PROGRAM MAIN
VAR_INPUT
   // Use an external Switch to start justify Offset/Gain
   bEnable AT%I*         :BOOL;
   PAI_Sample AT%I*      :DINT; // The linked Variable to the EL3751 Result
END_VAR
VAR
   // "Main" State controlling Offset/Gain adjusting:
   nMainCal_State        :BYTE:=0;
   // ===============================================
   // For CoE Object 0x8005 access:
   fb_coe_write          :FB_EcCoESdoWrite;
   
   // Enter your Net-Id here:
   userNetId             :T_AmsNetId := 'xxx.xx.1.1.2.1';
   // Enter your EL3751 adress here:
   userSlaveAddr         :UINT := 1001;
   
   wCoEIndexScaler       :WORD := 16#8005;
   bySubIndScalGain      :BYTE := 16#02;
   bySubIndScalOffs      :BYTE := 16#01;
   nADSErrId             :UDINT; // Copy of ADS-Error ID
   // ===============================================
   // Variables for calculation
   fb_get_min_max        :FB_GET_MIN_MAX;
   // Variables used for offset scaling:
   nSTATE_SCALE_OFFSET   :INT := 0;
   bStartScaleOffset     :BOOL := FALSE;
   bScaleOffsetDone      :BOOL := FALSE;
   fOffsetDeviationVal   :REAL;
   fScalerOffset_COE     :LREAL := 0;
   wOFFSET_MIN_VAL_REF   :WORD;
   // Variables used for gain scaling:
   nSTATE_SCALE_GAIN     :INT := 0;
   bStartScaleGain       :BOOL := FALSE;
   bScaleGainDone        :BOOL := FALSE;
   fScalerGain_COE       :REAL := 1;
   nPRESET_MAX_VAL       :DINT := 3000000; // Target amplitude value
   nMaxAmplVal           :DINT;
   // ===============================================
   // Variables for intermediate results
   nValue                :DINT; // Used for Offset (adding)
   fValue                :REAL; // Used for Gain (multiply)
END_VAR

// Example program 1 and 2 program code:
// =====================================
IF bEnable AND (nMainCal_State = 0) THEN // Poll Switch
   nMainCal_State := 10; // Start
END_IF
CASE nMainCal_State OF // Main-State Procedure
   10:
      bStartScaleOffset:=TRUE; // Start with Offset scaling
      wOFFSET_MIN_VAL_REF := 2000; // Prepare deviation tolerance value scope
      nMainCal_State := nMainCal_State + 1; // next state
   11:
      IF bScaleOffsetDone THEN
         bStartScaleGain := TRUE; // Continue with gain scaling
         nMainCal_State := nMainCal_State + 1;
      END_IF
   12:
      IF bScaleGainDone THEN
         nMainCal_State := nMainCal_State + 1; // all done
      END_IF
   13:
      IF NOT bEnable THEN
         nMainCal_State :=0; // Initalization for next start by user
      END_IF
END_CASE
// ----- Offset scaling -----
IF bStartScaleOffset THEN
   CASE nSTATE_SCALE_OFFSET OF
   0:
      bScaleOffsetDone := FALSE; // Initialization of confirmation flag
      nSTATE_SCALE_OFFSET := nSTATE_SCALE_OFFSET + 1;
   1:
      fb_get_min_max(nInputValue:=PAI_Sample); // Get min/max Values by current Sample value
      IF fb_get_min_max.bRESULT THEN // Wait if Limit-Values are valid
         fb_coe_write(bExecute := FALSE); // Prepare CoE access
         nSTATE_SCALE_OFFSET := nSTATE_SCALE_OFFSET + 1; // Min/Max Values valid - go to next state
      END_IF
   2:
      // Calculate current offset deviation
      fOffsetDeviationVal :=
      LREAL_TO_REAL(ABS(fb_get_min_max.nMinVal) - ((ABS(fb_get_min_max.nMaxVal) + ABS(fb_get_min_max.nMinVal))/2));
      // Offset deviation check:
      IF ABS(fOffsetDeviationVal) < wOFFSET_MIN_VAL_REF THEN
         // Deviation in acceptable range - offset scaling done
         bScaleOffsetDone := TRUE;
         bStartScaleOffset := FALSE;
         nSTATE_SCALE_OFFSET := 0;
      ELSE
         // Calculate new offset value (consider pre-assigned value)
         nValue := LREAL_TO_DINT(fScalerOffset_COE + fOffsetDeviationVal);
         // ..proceed zero-point shift: write value into CoE Object
         fb_coe_write(
            sNetId:= userNetId,
            nSlaveAddr:= userSlaveAddr,
            nSubIndex:= bySubIndScalOffs,
            nIndex:= wCoEIndexScaler,
            pSrcBuf:= ADR(nValue), // Offset-Value (CoE 0x8005:01)
            cbBufLen:= SIZEOF(nValue),
            bExecute:= TRUE,
            tTimeout:= T#1S,
            bBusy=> ,
            bError=> ,
            nErrId=> );
         nSTATE_SCALE_OFFSET := nSTATE_SCALE_OFFSET + 1;
      END_IF
   3:
      fb_coe_write();
      IF fb_coe_write.bError THEN
         nSTATE_SCALE_OFFSET := 100;
      ELSE
         IF NOT fb_coe_write.bBusy THEN
            fScalerOffset_COE := DINT_TO_LREAL(nValue);
            nSTATE_SCALE_OFFSET := 0;
         END_IF
      END_IF
   100:
      // Copy Error ID for interpretation:
      nADSErrId := fb_coe_write.nErrId;
   END_CASE
END_IF
// ----- Justify gain: write calculated value in CoE - Object 0x8005 -----
IF bStartScaleGain THEN
   CASE nSTATE_SCALE_GAIN OF
   0:
      bScaleGainDone := FALSE; // Initialization of confirmation flag
      nSTATE_SCALE_GAIN := nSTATE_SCALE_GAIN + 1;
   1:
      // Get min/max Values by current Sample value:
      fb_get_min_max(nInputValue:=PAI_Sample);
      IF fb_get_min_max.bRESULT THEN // Wait if Limit-Values are valid
         fb_coe_write(bExecute := FALSE); // Prepare CoE access
         nSTATE_SCALE_GAIN := nSTATE_SCALE_GAIN + 1; // Min/Max Values valid - go to next state
      END_IF
   2:
      // Get current amplitude for calculating the gain value:
      nMaxAmplVal := MAX(ABS(fb_get_min_max.nMaxVal), ABS(fb_get_min_max.nMinVal));
      // Avoid division by zero:
      IF nMaxAmplVal = 0 THEN
         nSTATE_SCALE_GAIN := 100;
      ELSE
         // Calculate Gain:
         fValue := DINT_TO_REAL(nPRESET_MAX_VAL)/DINT_TO_REAL(nMaxAmplVal) * fScalerGain_COE;
         // Shift gain value by 16 Bit left and convert to DINT:
         nValue := REAL_TO_DINT(fValue * 65536);
         // Write to CoE Index:
         fb_coe_write(
         sNetId:= userNetId,
         nSlaveAddr:= userSlaveAddr,
         nSubIndex:= bySubIndScalGain,
         nIndex:= wCoEIndexScaler,
         pSrcBuf:= ADR(nValue), // Gain-Value (CoE 0x8005:02)
         cbBufLen:= SIZEOF(nValue),
         bExecute:= TRUE,
         tTimeout:= T#1S,
         bBusy=> ,
         bError=> ,
         nErrId=> );
         nSTATE_SCALE_GAIN := nSTATE_SCALE_GAIN + 1;
      END_IF
   3:
      fb_coe_write();
      IF fb_coe_write.bError THEN
         nSTATE_SCALE_GAIN := 100;
      ELSE
         IF NOT fb_coe_write.bBusy THEN
            fScalerGain_COE := fValue;
            bStartScaleGain := FALSE; // gain scaling done
            bScaleGainDone := TRUE;
            nSTATE_SCALE_GAIN := 0; // Set initial state
         END_IF
      END_IF
   100:
      // Copy Error ID for interpretation:
      nADSErrId := fb_coe_write.nErrId;
   END_CASE
END_IF

END_PROGRAM
